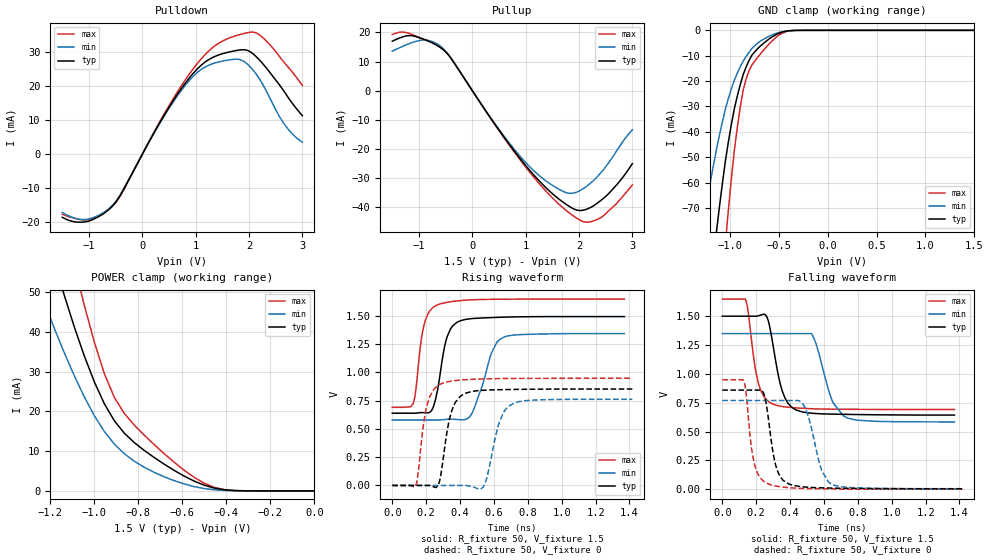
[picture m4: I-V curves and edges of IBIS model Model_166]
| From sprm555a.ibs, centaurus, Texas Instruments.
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| Model based on original model for BCSHTLTCSCDVPBFZ_SSGFV
|   Sub model SR00_10MA_10PER_1P5
[model]   Model_166
|[Description]  [1.5V-3-STATE-X-FASTEST:10MA, IND, 10%]
|   Fastest slew rate (SR[1:0] = "00"), 0.80 * RExt = 1.250 * Iout
|   (I[2:0] = "101"), 10mA nominal with Rext = 50R, ,Industrial
|   temperature range (-40C to 125C, 25C nominal),10% power supply
|   tolerance
|[Input Load]
|[Output Drive] FASTEST:10MA
|Voltage   1.5V
|Mode   3-STATE
Model_type   3-state
Polarity   Non-Inverting
Enable   Active-Low
Cref =  15pF
Rref =  100.0000M
Vref =  0V
Vmeas =  0.75
C_comp   1.865048p   1.676829p   1.989968p
[Temperature Range]   25   125   -40
[Voltage Range]   1.5   1.35   1.65
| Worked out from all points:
|   slope of the pulldown table from 0 to 0.225 V, typ, clamps not added: 34.7 ohm
|   slope of the pullup table from 0 to 0.225 V, typ, clamps not added: 36.1 ohm
|   GND clamp passes 1 mA (typ) near -0.49 V on its own axis
|   POWER clamp passes 1 mA (typ) near -0.47 V on its own axis
|   rising waveform, R_fixture 50, V_fixture 1.5: 20-80 % time 63.6ps typ, 96.3ps min, 52.5ps max; typ from 0.64 V to 1.5 V
|   rising waveform, R_fixture 50, V_fixture 0: 20-80 % time 62.2ps typ, 75.2ps min, 56.5ps max; typ from 0 V to 0.854 V
|   falling waveform, R_fixture 50, V_fixture 1.5: 20-80 % time 73.6ps typ, 94.1ps min, 61.8ps max; typ from 1.5 V to 0.643 V
|   falling waveform, R_fixture 50, V_fixture 0: 20-80 % time 57.1ps typ, 77.9ps min, 49.4ps max; typ from 0.86 V to 0.003 V
[POWER_clamp]
-1.5V     126mA      88.79mA    168.7mA
-1.242V   69.8mA     49.45mA    94.34mA
-1.136V   49.16mA    34.72mA    67.51mA
-1.061V   36.35mA    25.4mA     50.03mA
-1.045V   33.92mA    23.63mA    46.66mA
-954.5mV  21.93mA    14.95mA    29.5mA
-909.1mV  17.64mA    11.79mA    23.52mA
-863.6mV  14.51mA    9.351mA    19.47mA
-772.7mV  10.16mA    5.94mA     13.99mA
-590.9mV  3.705mA    1.741mA    5.166mA
-454.5mV  710.5uA    279.1uA    892.1uA
0V        1.424nA    14.34nA    3.127nA
[Pulldown]
-1.5V     -18.53mA   -17.11mA   -17.64mA
-1V       -19.61mA   -19mA      -19.13mA
-727.3mV  -17.47mA   -17.14mA   -17.24mA
-500mV    -14.14mA   -13.9mA    -14.19mA
272.7mV   7.805mA    7.637mA    8.027mA
681.8mV   18.19mA    17.72mA    18.92mA
1.045V    25.32mA    24.25mA    26.96mA
1.364V    28.79mA    26.85mA    31.92mA
1.818V    30.65mA    27.86mA    35.15mA
2.136V    28.67mA    23.53mA    35.66mA
2.636V    18.97mA    9.445mA    27.43mA
3V        11.34mA    3.552mA    20.22mA
[Pullup]
-1.5V     17mA       13.57mA    19.29mA
-1.136V   18.91mA    16.49mA    19.38mA
-863.6mV  17.34mA    17.39mA    17.41mA
-590.9mV  14.75mA    15.19mA    14.74mA
-409.1mV  11.37mA    11.41mA    11.41mA
909.1mV   -23.65mA   -22.84mA   -24.11mA
1.318V    -32.26mA   -30.18mA   -33.3mA
1.773V    -39.28mA   -35.15mA   -41.4mA
2.045V    -41.2mA    -34.1mA    -44.8mA
2.318V    -39.01mA   -30.07mA   -44.47mA
2.682V    -32.88mA   -21.38mA   -39.23mA
3V        -25.08mA   -13.45mA   -32.44mA
[GND_clamp]
-1.5V     -219.3mA   -131.6mA   -364.3mA
-1.288V   -134.4mA   -79.74mA   -225.6mA
-1.258V   -122.9mA   -72.77mA   -206.3mA
-1.136V   -79.27mA   -46.88mA   -132.4mA
-1.045V   -51.5mA    -31.06mA   -84.11mA
-1.015V   -44.02mA   -26.9mA    -70.91mA
-954.5mV  -31.01mA   -19.7mA    -47.55mA
-863.6mV  -17.48mA   -12.16mA   -23.55mA
-803mV    -11.81mA   -8.597mA   -15.85mA
-681.8mV  -5.986mA   -4.096mA   -9.026mA
-378.8mV  -126.2uA   -131.8uA   -179.7uA
1.5V      1.424nA    207.1nA    1.498nA
[Ramp]
dV/dt_f 0.52682893/74.097773p 0.47447032/94.213539p 0.58332352/61.634079p
dV/dt_r 0.52646484/63.076965p 0.47893326/75.596715p 0.57788609/56.374557p
R_load = 50
[Rising Waveform]
R_fixture = 50
V_fixture = 1.5
V_fixture_min = 1.35
V_fixture_max = 1.65
0s        639.6mV    579.9mV    691.6mV
123.1ps   639.6mV    579.9mV    723.8mV
187.2ps   644.5mV    579.9mV    1.42V
231.2ps   661.2mV    579.9mV    1.562V
265.7ps   834.8mV    579.9mV    1.598V
324.2ps   1.318V     585.7mV    1.621V
401.2ps   1.457V     581.9mV    1.637V
472.9ps   1.477V     647mV      1.643V
634.9ps   1.489V     1.293V     1.648V
1.37ns    1.495V     1.344V     1.65V
[Rising Waveform]
R_fixture = 50
V_fixture = 0
V_fixture_min = 0
V_fixture_max = 0
0s        0V         0V         0V
137.8ps   0V         0V         -5.401mV
200ps     0V         0V         677.6mV
285.4ps   83.89mV    0V         898mV
348.9ps   651mV      0V         923.9mV
424.5ps   811.1mV    0V         935.5mV
536.2ps   842.4mV    -15.3mV    942.7mV
630.4ps   847.6mV    553.3mV    945.9mV
718.7ps   849.9mV    728.9mV    947.3mV
1.417ns   853.5mV    762.7mV    949.2mV
[Falling Waveform]
R_fixture = 50
V_fixture = 1.5
V_fixture_min = 1.35
V_fixture_max = 1.65
0s        1.501V     1.35V      1.649V
136.8ps   1.501V     1.35V      1.649V
208.2ps   1.502V     1.35V      949.4mV
262.4ps   1.498V     1.35V      773.9mV
295.2ps   1.287V     1.35V      741mV
353.3ps   854.6mV    1.35V      717.3mV
438.7ps   685.2mV    1.35V      704.8mV
535.3ps   658mV      1.327V     697.4mV
715.3ps   649.2mV    634.9mV    693.2mV
1.37ns    642.9mV    583.5mV    690.8mV
[Falling Waveform]
R_fixture = 50
V_fixture = 0
V_fixture_min = 0
V_fixture_max = 0
0s        859.5mV    768.9mV    948.9mV
130ps     859.5mV    768.9mV    927.6mV
188.8ps   859.5mV    768.9mV    224.4mV
243.6ps   833.7mV    768.9mV    69.1mV
270.8ps   627.5mV    768.9mV    45.93mV
316.6ps   201mV      768.9mV    26.68mV
392.4ps   45.27mV    768.9mV    13.19mV
483.5ps   19.2mV     721.1mV    6.093mV
646.9ps   9.34mV     42.11mV    2.142mV
1.417ns   3.35mV     4.187mV    0V
